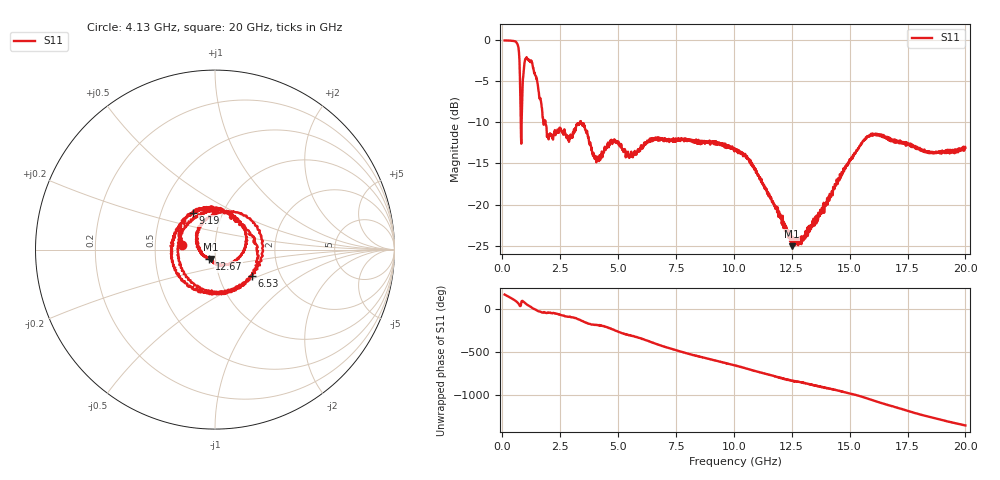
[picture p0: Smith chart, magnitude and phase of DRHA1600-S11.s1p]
!Keysight Technologies,P9374A,MY57211922,A.15.40.13
!Date: Wednesday, August 05, 2026 12:12:22
!Correction: S11(C  1-Port  )
!S1P File: Measurement: S11:
# Hz S  dB  R 50
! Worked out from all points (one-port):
!   1991 points, 100 MHz to 20 GHz, reference 50 ohm
!   lowest |S11| = -25.1 dB at 12.5 GHz (marker M1), VSWR 1.12, Z = 47.7 - j4.95 ohm
!   |S11| at or under -10 dB: 798.5 MHz to 835.5 MHz (37.01 MHz wide, 4.53 % of centre); 1.865 GHz to 3.365 GHz (1.501 GHz wide, 57.4 % of centre); 3.399 GHz to end of sweep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
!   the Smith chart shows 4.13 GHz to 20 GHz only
!   S11 on the Smith chart (normalised r, x): 4.13 GHz: 0.69, +0.04; 6.53 GHz: 1.43, -0.45; 9.19 GHz: 0.72, +0.31; 12.67 GHz: 0.93, -0.10; 20 GHz: 0.91, +0.42
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1e8  -0.02 165.8
3.3e8  -0.04 132.6
5.6e8  -0.12 95.0
6.9e8  -0.80 64.2
8e8  -10.26 38.3
9e8  -4.54 84.7
1e9  -2.31 63.1
1.23e9  -2.58 23.9
1.59e9  -6.80 -30.3
2e9  -12.06 -42.4
2.59e9  -11.19 -75.0
3.52e9  -10.44 -149.5
4.13e9  -14.53 171.9
5.08e9  -12.59 88.1
6.53e9  -11.99 -35.5
7.57e9  -12.08 -124.2
8.28e9  -12.47 -177.5
9.19e9  -12.44 121.0
1.005e10  -13.26 63.8
1.134e10  -18.05 -28.7
1.25e10  -25.07 -111.9
1.254e10  -23.95 -114.4
1.267e10  -24.28 -120.5
1.503e10  -14.47 99.7
1.626e10  -11.48 -1.6
1.752e10  -12.51 -103.3
1.865e10  -13.63 174.5
2e10  -13.09 89.5
